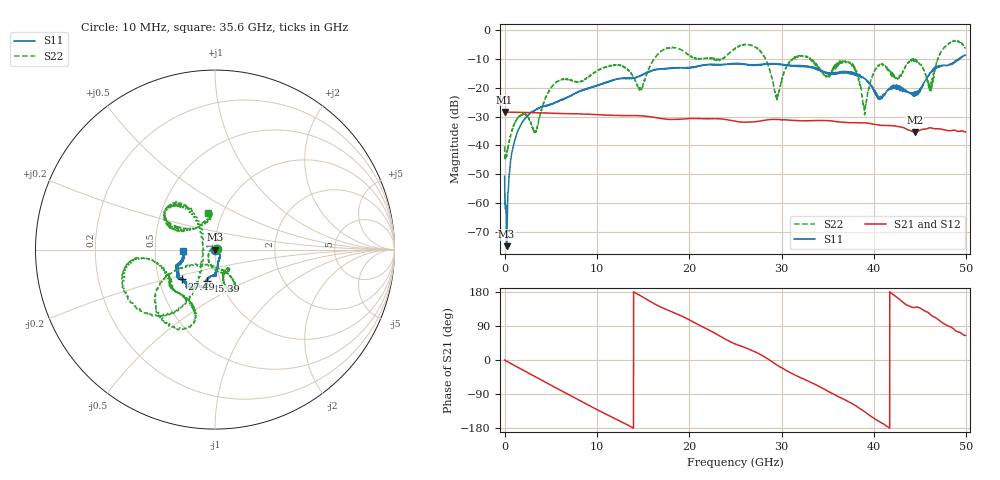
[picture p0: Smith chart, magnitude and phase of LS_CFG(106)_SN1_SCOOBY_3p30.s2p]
!Keysight Technologies,N5245B,MY58422026,A.13.80.08
!Date: Friday, March 20, 2020 00:00:25
!Correction: S11(Full 2 Port(1,2))
!S21(Full 2 Port(1,2))
!S12(Full 2 Port(1,2))
!S22(Full 2 Port(1,2))
!S2P File: Measurements: S11, S21, S12, S22:
# Hz S DB R 50.0
!freq dBS11 angS11 dBS21 angS21 dBS12 angS12 dBS22 angS22
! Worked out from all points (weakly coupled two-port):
!   4991 points, 10 MHz to 49.91 GHz, reference 50 ohm
!   highest |S21| = -28.44 dB at 10 MHz (marker M1); lowest = -35.5 dB at 44.43 GHz (marker M2)
!   lowest |S11| = -74.8 dB at 230 MHz (marker M3), VSWR 1.00, Z = 50 + j0.0182 ohm
!   |S11| at or under -10 dB: start of sweep to 49.24 GHz; 49.29274 GHz to 49.33672 GHz (43.98 MHz wide, 0.0892 % of centre)
!   |S22| runs from -44.6 to -3.7 dB; largest |S21 - S12| = 0.00037
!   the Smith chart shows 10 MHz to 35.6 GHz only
!   S11 on the Smith chart (normalised r, x): 10 MHz: 1.00, -0.01; 15.39 GHz: 0.86, -0.31; 27.49 GHz: 0.66, -0.23; 35.6 GHz: 0.70, -0.02
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1e7  -50.58 -106.7  -28.44 -0.3  -28.43 -0.3  -40.30 5.2
2.3e8  -74.80 87.6  -28.48 -3.2  -28.46 -3.2  -43.47 -45.6
8.6e8  -41.35 -37.1  -28.51 -11.6  -28.50 -11.6  -34.17 -39.6
2.01e9  -31.56 -41.5  -28.58 -26.8  -28.57 -26.7  -29.07 13.7
3.31e9  -27.71 -50.0  -28.68 -43.8  -28.67 -43.7  -35.24 130.4
5.37e9  -25.22 -63.2  -28.86 -71.0  -28.86 -71.0  -18.84 -88.4
8.33e9  -21.15 -79.7  -29.12 -109.4  -29.12 -109.3  -17.80 -63.8
1.539e10  -14.77 -104.6  -29.91 159.8  -29.90 159.8  -15.51 -146.3
1.665e10  -13.69 -104.9  -30.52 143.0  -30.50 143.0  -8.28 -145.6
2.496e10  -11.76 -127.4  -31.57 42.5  -31.56 42.7  -6.55 -170.9
2.749e10  -12.19 -138.2  -31.65 17.3  -31.65 17.6  -6.66 -127.8
2.947e10  -11.73 -142.8  -31.01 -12.6  -30.99 -12.3  -23.33 -175.7
3.328e10  -12.96 -159.0  -31.42 -60.4  -31.42 -60.0  -10.60 153.1
3.56e10  -14.91 -176.2  -31.63 -90.0  -31.57 -89.6  -13.88 101.5
3.77e10  -15.46 174.4  -32.11 -115.9  -32.04 -116.1  -12.17 131.5
3.902e10  -16.86 172.9  -32.16 -136.8  -32.15 -137.0  -28.62 -113.6
4.021e10  -22.48 162.6  -32.76 -156.9  -32.74 -157.0  -13.43 -8.7
4.16e10  -20.38 101.9  -33.10 -178.1  -33.12 -178.0  -14.11 22.5
4.443e10  -22.75 48.5  -35.49 138.9  -35.53 139.3  -10.71 -18.6
4.614e10  -14.81 3.6  -33.90 119.6  -33.91 119.8  -21.36 -50.8
4.757e10  -12.26 4.8  -34.56 96.0  -34.56 96.0  -6.26 -80.3
4.991e10  -8.80 -13.9  -35.33 64.7  -35.35 64.7  -6.28 -28.7
